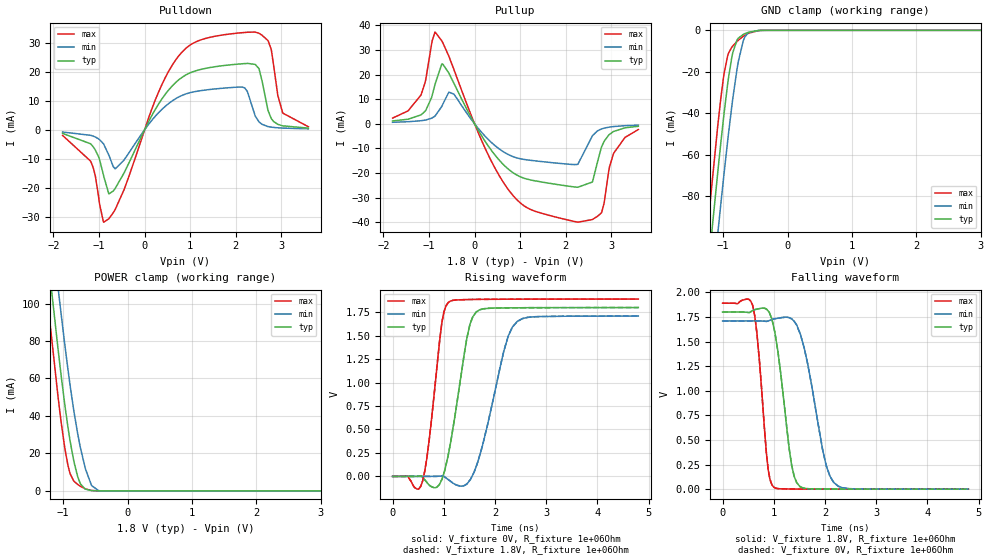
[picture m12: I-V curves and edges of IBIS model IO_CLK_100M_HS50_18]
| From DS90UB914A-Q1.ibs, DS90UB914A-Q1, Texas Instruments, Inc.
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|   Model IO_CLK_100M_HS50_18
[Model]   IO_CLK_100M_HS50_18
Model_type   I/O
Polarity   Non-Inverting
Enable   Active-Low
Vinl = 0.63
Vinh = 1.17
Vmeas = 0.9
Vref = 1.8
Cref = 1pF
Rref = 1000000
|   typ   min   max
C_comp   1.107pF   1.107pF   1.107pF
[Voltage Range]   1.8   1.71   1.89
[Temperature Range]   25   105   -40
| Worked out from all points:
|   slope of the pulldown table from 0 to 0.27 V, typ, clamps not added: 34 ohm
|   slope of the pullup table from 0 to 0.27 V, typ, clamps not added: 33 ohm
|   GND clamp passes 1 mA (typ) near -0.61 V on its own axis
|   POWER clamp passes 1 mA (typ) near -0.66 V on its own axis
|   falling waveform, V_fixture 1.8V, R_fixture 1e+06Ohm: 20-80 % time 248ps typ, 357ps min, 171ps max; typ from 1.8 V to 0 V
|   rising waveform, V_fixture 0V, R_fixture 1e+06Ohm: 20-80 % time 308ps typ, 428ps min, 221ps max; typ from 0 V to 1.8 V
|   rising waveform, V_fixture 1.8V, R_fixture 1e+06Ohm: 20-80 % time 308ps typ, 428ps min, 221ps max; typ from 0 V to 1.8 V
|   falling waveform, V_fixture 0V, R_fixture 1e+06Ohm: 20-80 % time 248ps typ, 357ps min, 171ps max; typ from 1.8 V to 0 V
[Pulldown]
|   Voltage   I(typ)   I(min)   I(max)
-1.8V     -1.226mA   -753.5uA   -1.919mA
-1.184V   -4.802mA   -1.886mA   -10.78mA
-898.2mV  -15.9mA    -4.902mA   -31.82mA
-784.8mV  -22.07mA   -8.667mA   -30.64mA
-644.4mV  -20.17mA   -13.45mA   -27.42mA
721.8mV   16.86mA    11.08mA    24.9mA
2.266V    22.88mA    12.74mA    33.63mA
2.509V    21.12mA    2.791mA    33.28mA
2.714V    6.495mA    1.113mA    30.6mA
2.828V    2.927mA    837.2uA    22.72mA
3.033V    1.373mA    595uA      5.772mA
3.595V    587.1uA    345.6uA    1.067mA
[GND Clamp]
|   Voltage   I(typ)   I(min)   I(max)
-1.8V     -305.9mA   -328.3mA   -290.1mA
-1.233V   -115.7mA   -144.4mA   -93.47mA
-1.174V   -96.56mA   -125.8mA   -74.01mA
-1.087V   -69.56mA   -99.16mA   -47.1mA
-1.039V   -55.02mA   -84.55mA   -33.4mA
-984.6mV  -39.77mA   -68.76mA   -20.69mA
-930.6mV  -26.08mA   -53.61mA   -12.4mA
-865.8mV  -13.1mA    -36.71mA   -8.15mA
-763.2mV  -3.75mA    -14.91mA   -4.764mA
-687.6mV  -1.977mA   -5.052mA   -2.868mA
-450mV    -68.15uA   -51.16uA   -140.3uA
3.595V    0A         0A         0A
[Pullup]
|   Voltage   I(typ)   I(min)   I(max)
-1.8V     1.154mA    611.9uA    2.3mA
-1.179V   3.59mA     1.23mA     11.6mA
-865.8mV  16.16mA    3.164mA    37.25mA
-698.4mV  24.28mA    7.889mA    32.97mA
-450mV    16.32mA    11.98mA    21.87mA
230.4mV   -7.097mA   -5.029mA   -9.913mA
759.6mV   -18.7mA    -12.67mA   -27.19mA
2.266V    -25.78mA   -16.48mA   -39.98mA
2.585V    -23.67mA   -4.951mA   -38.92mA
2.779V    -9.835mA   -2.149mA   -36.3mA
3.049V    -3.154mA   -1.133mA   -12.14mA
3.595V    -1.016mA   -567.4uA   -2.336mA
[POWER Clamp]
|   Voltage   I(typ)   I(min)   I(max)
-1.8V     314.3mA    339.7mA    296mA
-1.454V   197.1mA    226.6mA    174.7mA
-1.222V   120.5mA    152.5mA    95.53mA
-1.201V   113.5mA    145.7mA    88.4mA
-1.082V   76.47mA    109.3mA    50.98mA
-1.044V   65.28mA    98.08mA    40.18mA
-898.2mV  27.99mA    57.89mA    10.03mA
-774mV    7.614mA    30.49mA    3.452mA
-660.6mV  1.08mA     12.7mA     1.21mA
-558mV    201.4uA    2.857mA    238.7uA
-433.8mV  12.45uA    107uA      11.31uA
3.595V    0A         0A         0A
[Ramp]
R_load = 1e+06
|   typ   min   max
dV/dt_r   1.0799/3.0752e-10   1.02561/4.28255e-10   1.13396/2.21232e-10
dV/dt_f   1.07991/2.47873e-10   1.02566/3.57252e-10   1.13397/1.70612e-10
[Falling Waveform]
V_fixture = 1.8V
V_fixture_min = 1.71V
V_fixture_max = 1.89V
R_fixture = 1e+06Ohm
C_fixture = 0F
|   Time   V(typ)   V(min)   V(max)
0s        1.8V       1.71V      1.89V
588.6ps   1.816V     1.71V      1.867V
670.7ps   1.829V     1.71V      1.585V
889.8ps   1.811V     1.709V     203.6mV
1.002ns   1.639V     1.73V      19.16mV
1.35ns    240.7mV    1.731V     1.567mV
1.512ns   26.42mV    1.585V     1.12mV
1.954ns   1.809mV    402.4mV    581.5uV
2.171ns   1.396mV    68.4mV     316.8uV
4.8ns     69.96uV    162.9uV    39.36uV
[Rising Waveform]
V_fixture = 0V
V_fixture_min = 0V
V_fixture_max = 0V
R_fixture = 1e+06Ohm
C_fixture = 0F
|   Time   V(typ)   V(min)   V(max)
0s        12.21uV    69.8uV     5.712uV
588.6ps   -11.33mV   19.58uV    -45.74mV
718.9ps   -94.45mV   8.465uV    403.1mV
963.5ps   -32.35mV   4.033mV    1.64V
1.088ns   230.3mV    -34.5mV    1.853V
1.449ns   1.468V     -82.07mV   1.885V
1.633ns   1.752V     105.6mV    1.886V
2.171ns   1.795V     1.331V     1.888V
2.436ns   1.797V     1.652V     1.889V
4.8ns     1.8V       1.709V     1.89V
[Rising Waveform]
V_fixture = 1.8V
V_fixture_min = 1.71V
V_fixture_max = 1.89V
R_fixture = 1e+06Ohm
C_fixture = 0F
|   Time   V(typ)   V(min)   V(max)
0s        66.79uV    148.3uV    45.03uV
588.6ps   -11.27mV   97.7uV     -45.4mV
718.9ps   -94.3mV    86.51uV    403.6mV
963.5ps   -31.93mV   4.11mV     1.64V
1.088ns   230.8mV    -34.39mV   1.854V
1.449ns   1.469V     -81.62mV   1.885V
1.633ns   1.752V     106.2mV    1.886V
2.171ns   1.795V     1.332V     1.888V
2.436ns   1.797V     1.652V     1.889V
4.8ns     1.8V       1.71V      1.89V
[Falling Waveform]
|Gnd
V_fixture = 0V
V_fixture_min = 0V
V_fixture_max = 0V
R_fixture = 1e+06Ohm
C_fixture = 0F
|   Time   V(typ)   V(min)   V(max)
0s        1.8V       1.71V      1.89V
588.6ps   1.816V     1.71V      1.867V
670.7ps   1.829V     1.71V      1.584V
889.8ps   1.811V     1.709V     203.4mV
1.002ns   1.639V     1.73V      19.08mV
1.35ns    240.4mV    1.73V      1.52mV
1.512ns   26.3mV     1.585V     1.075mV
1.954ns   1.742mV    401.9mV    539.5uV
2.171ns   1.331mV    68.18mV    276.1uV
4.8ns     15.35uV    84.22uV    55.9nV
